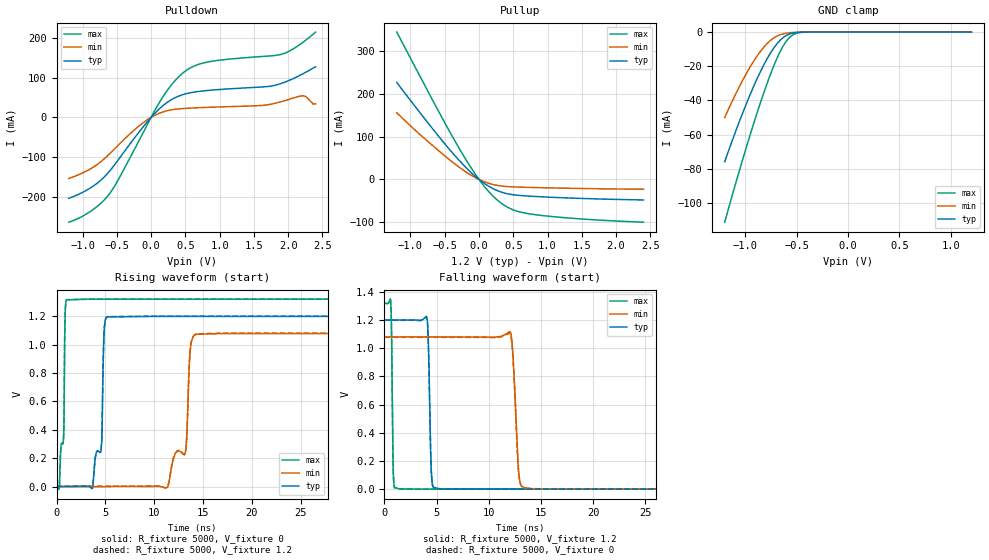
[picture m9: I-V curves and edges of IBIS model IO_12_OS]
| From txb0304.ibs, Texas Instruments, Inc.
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[Model]   IO_12_OS
Model_type  I/O
Vinl=0.378
Vinh=0.858
Enable   Active-High
Vref =   0
Rref =   5000
Cref =   15p
Vmeas =   0.6
| variable   typ   min   max
C_comp   3.93pF   3.64pF   4.13pF
| C_pullup   7.73pF   4.75pF   9.19pF
| C_pulldown   8.78pF   3.51pF   11.19pF
| C_tri-state   3.93pF   3.64pF   4.13pF
[Temperature Range]   40   100   -40
| Ambient temperature   25   85   -40
[Voltage range]   1.2   1.08   1.32
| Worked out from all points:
|   slope of the pulldown table from 0 to 0.18 V, typ, clamps not added: 5.89 ohm
|   slope of the pullup table from 0 to 0.18 V, typ, clamps not added: 9.36 ohm
|   GND clamp passes 1 mA (typ) near -0.56 V on its own axis
|   rising waveform, R_fixture 5000, V_fixture 0: 20-80 % time 352ps typ, 1.54ns min, 403ps max; typ from 0 V to 1.2 V
|   falling waveform, R_fixture 5000, V_fixture 1.2: 20-80 % time 202ps typ, 401ps min, 121ps max; typ from 1.2 V to 0.001 V
|   rising waveform, R_fixture 5000, V_fixture 1.2: 20-80 % time 359ps typ, 1.54ns min, 403ps max; typ from 0.001 V to 1.2 V
|   falling waveform, R_fixture 5000, V_fixture 0: 20-80 % time 202ps typ, 402ps min, 121ps max; typ from 1.2 V to 0 V
[GND Clamp]
| IO_12B
|   Voltage   I(typ)   I(min)   I(max)
-1.2V     -75.93mA   -50.03mA   -111.3mA
-1.09V    -57.58mA   -35.88mA   -87.94mA
-990mV    -42.07mA   -24.33mA   -67.55mA
-900mV    -29.33mA   -15.35mA   -50.15mA
-820mV    -19.29mA   -8.867mA   -35.65mA
-740mV    -10.89mA   -4.215mA   -22.43mA
-670mV    -5.38mA    -1.799mA   -12.58mA
-610mV    -2.329mA   -749.6uA   -6.159mA
-555mV    -857.1uA   -301.9uA   -2.435mA
-495mV    -231uA     -94.89uA   -625.1uA
-400mV    -20.35uA   -9.848uA   -38.49uA
1.2V      331.9pA    31.51nA    21.6pA
[Pulldown]
| IO_12B
|   Voltage   I(typ)   I(min)   I(max)
-1.2V     -204.3mA   -154.3mA   -264.7mA
-870mV    -176.5mA   -128.5mA   -235.7mA
-615mV    -137.5mA   -93.64mA   -194.7mA
-460mV    -102.7mA   -66.96mA   -151.4mA
-10mV     -2.001mA   -1.036mA   -3.338mA
240mV     38.34mA    16.99mA    69mA
485mV     58.46mA    22.49mA    114.8mA
850mV     68.22mA    25.42mA    140.5mA
1.61V     76.6mA     29.98mA    153.5mA
1.91V     86.29mA    40.1mA     159.6mA
2.22V     110.5mA    54.35mA    190mA
2.4V      127.8mA    33.91mA    215.2mA
[Pullup]
| IO_12B
|   Voltage   I(typ)   I(min)   I(max)
-1.2V     226mA      155.1mA    343.1mA
-880mV    159.2mA    107.2mA    245.8mA
-570mV    96.74mA    64.38mA    152.6mA
-210mV    30.89mA    19.55mA    51.19mA
-65mV     8.697mA    5.275mA    14.88mA
65mV      -7.776mA   -4.5mA     -13.72mA
190mV     -20.09mA   -11.11mA   -36.43mA
310mV     -28.56mA   -14.93mA   -53.51mA
515mV     -35.95mA   -17.4mA    -71.79mA
795mV     -39.4mA    -18.77mA   -81.47mA
1.47V     -44.04mA   -20.94mA   -91.71mA
2.4V      -47.77mA   -22.8mA    -99.5mA
[Ramp]
| IO_12B
| variable   typ   min   max
dV/dt_r   0.73/7.78E-10   0.65/1.59E-09   0.80/4.19E-10
dV/dt_f   0.73/2.12E-10   0.67/4.23E-10   0.81/1.30E-10
R_load = 5000
[Rising Waveform]
| IO_12B
R_fixture =   5000
C_fixture =   0
L_fixture =   0
V_fixture =   0
V_fixture_min = 0
V_fixture_max = 0
|   Time   V(typ)   V(min)   V(max)
0s        1.499nV    13.85nV    110.7pV
705ps     164.7nV    13.84nV    327.5mV
1.027ns   207.6nV    13.84nV    1.315V
3.673ns   -12.88mV   3.658nV    1.319V
4.583ns   273.9mV    133.3nV    1.319V
5.185ns   1.194V     173.5nV    1.319V
11.36ns   1.198V     -4.4mV     1.319V
13.22ns   1.198V     250.1mV    1.319V
14.29ns   1.198V     1.072V     1.319V
65.37ns   1.198V     1.077V     1.319V
[Falling Waveform]
| IO_12B
R_fixture =   5000
C_fixture =   0
L_fixture =   0
V_fixture =   1.2
V_fixture_min = 1.08
V_fixture_max = 1.32
|   Time   V(typ)   V(min)   V(max)
0s        1.2V       1.08V      1.32V
607ps     1.2V       1.08V      1.317V
831ps     1.2V       1.08V      175.4mV
1.013ns   1.2V       1.08V      9.064mV
4.051ns   1.22V      1.08V      797.4uV
4.513ns   103.8mV    1.08V      795.1uV
5.003ns   6.779mV    1.08V      793.8uV
12.06ns   1.21mV     1.115V     790.9uV
13.5ns    1.209mV    8.971mV    790.9uV
65.37ns   1.204mV    2.118mV    790.8uV
[Rising Waveform]
| IO_12B
R_fixture =   5000
C_fixture =   0
L_fixture =   0
V_fixture =   1.2
V_fixture_min = 1.08
V_fixture_max = 1.32
|   Time   V(typ)   V(min)   V(max)
0s        1.204mV    2.118mV    790.8uV
705ps     1.205mV    2.118mV    328.8mV
1.027ns   1.205mV    2.118mV    1.316V
3.673ns   -11.68mV   2.118mV    1.32V
4.583ns   276.1mV    2.118mV    1.32V
5.185ns   1.196V     2.118mV    1.32V
11.35ns   1.2V       -3.963mV   1.32V
13.21ns   1.2V       249.4mV    1.32V
14.29ns   1.2V       1.075V     1.32V
65.37ns   1.2V       1.08V      1.32V
[Falling Waveform]
| IO_12B
R_fixture =   5000
C_fixture =   0
L_fixture =   0
V_fixture =   0
V_fixture_min = 0
V_fixture_max = 0
|   Time   V(typ)   V(min)   V(max)
0s        1.198V     1.077V     1.319V
607ps     1.198V     1.077V     1.315V
831ps     1.198V     1.077V     172.9mV
1.013ns   1.198V     1.077V     8.196mV
4.051ns   1.217V     1.077V     6.576uV
4.513ns   99.45mV    1.077V     4.258uV
5.003ns   5.489mV    1.077V     2.931uV
12.04ns   5.679uV    1.103V     88.92nV
13.47ns   4.402uV    6.911mV    58.86nV
65.37ns   3.807nV    279.2nV    4.735nV
